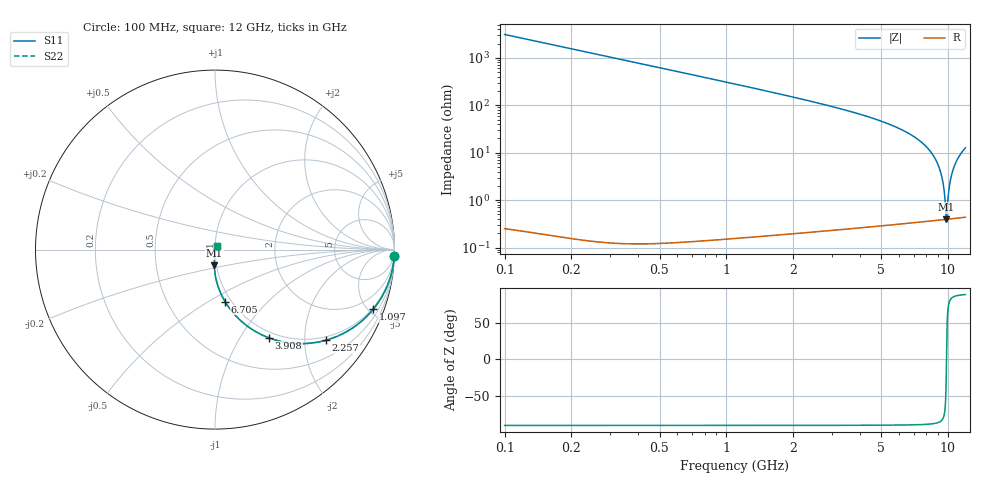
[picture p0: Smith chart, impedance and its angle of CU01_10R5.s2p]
! S-parameter model data by Modelithics Inc. support@modelithics.com 813-866-6335 Tampa FL USA
! S-Parameter data specifications:
! Substrate: 20-mil Rogers, substrate thickness, H=0.508mm, Dielectric constant, Er=3.75
! PCB Mounting Pad Footprint: Pad width, PadW=0.35mm , Pad length, PadL=0.30mm , Pad gap, PadG (edge-to-edge)=0.25mm , Reference planes=0.85mm apart
! Created Tue May  8 14:01:25 2018
# hz S ma R 50
! 2 Port Network Data from SP1.SP block
! freq  magS11  angS11  magS21  angS21  magS12  angS12  magS22  angS22
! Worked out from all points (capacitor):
!   801 points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, 100 MHz to 12 GHz, reference 50 ohm
!   read as one part in series: C = 512 fF near 159.5 MHz
!   lowest |Z| = 394 mohm at 9.858 GHz (marker M1)
!   series resonance near 9.859 GHz, so ESL is about 510 pH
!   S11 on the Smith chart (normalised r, x): 100 MHz: 1, -59; 1.097 GHz: 0.90, -5.33; 2.257 GHz: 0.91, -2.52; 3.908 GHz: 0.91, -1.34; 6.705 GHz: 0.94, -0.60; 12 GHz: 1.02, +0.04
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1e8  0.9995 -1.9  0.03217 88.1  0.03217 88.1  0.9995 -1.9
2.63625e8  0.9964 -5.1  0.08458 84.9  0.08458 84.9  0.9964 -5.1
4.42125e8  0.99 -8.6  0.1411 81.4  0.1411 81.4  0.99 -8.6
7.2475e8  0.9736 -13.9  0.2279 76.1  0.2279 76.1  0.9736 -13.9
1.096625e9  0.9419 -20.7  0.3353 69.3  0.3353 69.3  0.9419 -20.7
2.09325e9  0.8203 -36.9  0.5707 53.0  0.5707 53.0  0.8203 -36.9
2.256875e9  0.7978 -39.3  0.6017 50.6  0.6017 50.6  0.7978 -39.3
3.908e9  0.5761 -58.6  0.8152 31.2  0.8152 31.2  0.5761 -58.6
4.071625e9  0.5562 -60.1  0.8288 29.7  0.8288 29.7  0.5562 -60.1
6.05e9  0.3509 -75.1  0.9334 14.4  0.9334 14.4  0.3509 -75.1
6.7045e9  0.2957 -79.0  0.9521 10.4  0.9521 10.4  0.2957 -79.0
8.04325e9  0.1974 -85.8  0.9768 3.2  0.9768 3.2  0.1974 -85.8
9.858e9  0.08697 -92.5  0.9922 -5.0  0.9922 -5.0  0.08697 -92.5
1.002162e10  0.07801 -92.8  0.9929 -5.7  0.9929 -5.7  0.07801 -92.8
1.060175e10  0.04734 -93.2  0.9947 -8.0  0.9947 -8.0  0.04734 -93.2
1.101825e10  0.02636 -90.7  0.9954 -9.7  0.9954 -9.7  0.02636 -90.7
1.127112e10  0.01419 -83.6  0.9956 -10.7  0.9956 -10.7  0.01419 -83.6
1.149425e10  0.005037 -44.9  0.9956 -11.5  0.9956 -11.5  0.005037 -44.9
1.153888e10  0.004261 -20.2  0.9956 -11.7  0.9956 -11.7  0.004261 -20.2
1.159838e10  0.004764 15.6  0.9956 -11.9  0.9956 -11.9  0.004764 15.6
1.183638e10  0.01409 59.6  0.9955 -12.8  0.9955 -12.8  0.01409 59.6
1.2e10  0.02146 65.1  0.9953 -13.4  0.9953 -13.4  0.02146 65.1
